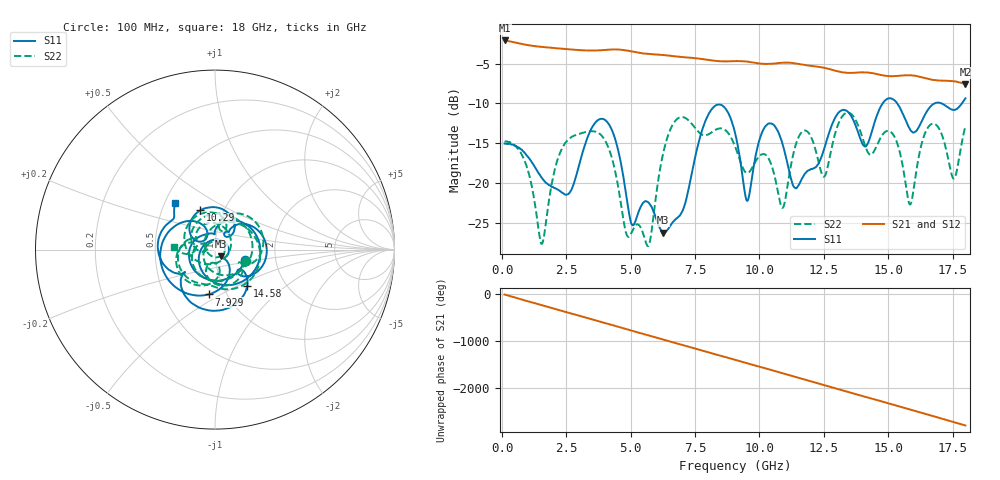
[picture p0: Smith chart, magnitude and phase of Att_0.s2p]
#  HZ  S  DB  R  50.00
! Rohde & Schwarz Vector Network Analyzer
! Rohde-Schwarz,ZNB40-4Port,1311601084101679,3.45
! Created: UTC 4/25/2025, 8:40:28 AM
! freq[Hz]  db:S11  ang:S11  db:S21  ang:S21  db:S12  ang:S12  db:S22  ang:S22
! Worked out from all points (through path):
!   1750 points, 100 MHz to 18 GHz, reference 50 ohm
!   highest |S21| = -2.12 dB at 100 MHz (marker M1); lowest = -7.6 dB at 18 GHz (marker M2)
!   group delay of S21, straight-line fit = 428 ps
!   lowest |S11| = -26.1 dB at 6.251 GHz (marker M3), VSWR 1.10, Z = 53.2 - j3.97 ohm
!   |S11| at or under -10 dB: start of sweep to 14.78 GHz; 15.35 GHz to 16.8 GHz (1.448 GHz wide, 9 % of centre); 17.08 GHz to 17.86 GHz (779.7 MHz wide, 4.46 % of centre)
!   |S22| runs from -27.8 to -11.1 dB; largest |S21 - S12| = 0.0012
!   S11 on the Smith chart (normalised r, x): 100 MHz: 1.39, -0.17; 7.929 GHz: 0.83, -0.44; 10.29 GHz: 0.78, +0.36; 14.58 GHz: 1.30, -0.57; 18 GHz: 0.57, +0.33
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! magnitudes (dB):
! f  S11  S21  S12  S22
! 100 MHz  -15.0  -2.1  -2.1  -14.7
! 1.543 GHz  -19.3  -2.9  -2.9  -27.6
! 2.208 GHz  -20.9  -3.1  -3.1  -16.5
! 3.088 GHz  -16.6  -3.3  -3.3  -13.7
! 4.071 GHz  -12.3  -3.3  -3.3  -15.1
! 4.9 GHz  -23.1  -3.4  -3.4  -26.7
! 5.698 GHz  -22.4  -3.8  -3.8  -27.7
! 6.067 GHz  -25.1  -3.9  -3.9  -19.6
! 6.251 GHz  -26.1  -3.9  -3.9  -16.4
! 7.929 GHz  -12.0  -4.5  -4.5  -14.0
! 9.055 GHz  -13.7  -4.7  -4.7  -15.4
! 9.526 GHz  -22.2  -4.8  -4.8  -18.7
! 10.29 GHz  -12.6  -5.1  -5.1  -16.6
! 10.9 GHz  -15.1  -4.9  -4.9  -23.1
! 12.04 GHz  -18.2  -5.3  -5.3  -14.5
! 12.49 GHz  -15.9  -5.5  -5.5  -19.2
! 14.58 GHz  -11.3  -6.3  -6.3  -15.1
! 15.02 GHz  -9.4  -6.6  -6.6  -13.4
! 15.85 GHz  -13.3  -6.5  -6.5  -22.6
! 16.57 GHz  -10.7  -6.9  -6.9  -12.9
! 17.55 GHz  -10.8  -7.2  -7.2  -19.4
! 18 GHz  -9.4  -7.6  -7.6  -12.9
